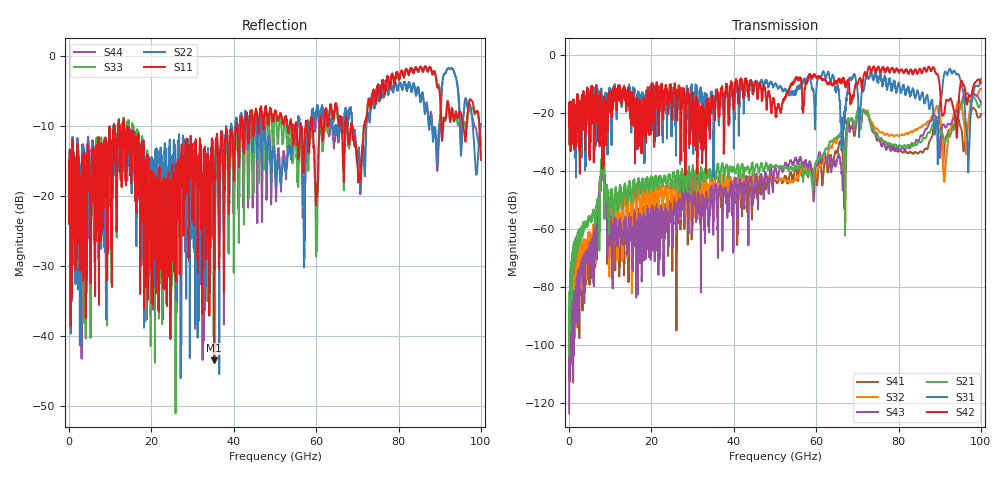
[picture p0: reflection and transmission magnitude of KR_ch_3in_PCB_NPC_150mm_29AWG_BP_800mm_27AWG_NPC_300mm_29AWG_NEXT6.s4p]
# GHz S RI R 45
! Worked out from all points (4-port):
!   4000 points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, 25 MHz to 100 GHz, reference 45 ohm
!   strongest paths, dB at 25 MHz, 25.02 GHz, 50.02 GHz, 75.03 GHz, 100 GHz:
!     S42: -21.3, -17.5, -18.0, -4.3, -9.8
!     S31: -21.3, -21.0, -10.2, -8.9, -8.4
!     S21: -103.8, -43.7, -38.2, -28.3, -17.0
!     S43: -123.6, -58.5, -39.1, -29.6, -16.4
!     S32: -108.9, -53.0, -42.7, -25.9, -11.9
!     S41: -111.4, -67.8, -43.2, -28.0, -20.5
!   lowest |S11| = -43.5 dB at 35.27 GHz (marker M1), VSWR 1.01, Z = 44.4 - j0.0041 ohm
!   |S11| at or under -10 dB: start of sweep to 10.87 GHz; 14.28 GHz to 40.62 GHz (26.34 GHz wide, 96 % of centre); 68.67 GHz to 71.56 GHz (2.899 GHz wide, 4.14 % of centre)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
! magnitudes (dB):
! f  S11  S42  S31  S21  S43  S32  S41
! 25 MHz  -16.8  -21.3  -21.3  -103.8  -123.6  -108.9  -111.4
! 8.025 GHz  -24.3  -27.6  -21.1  -40.7  -37.8  -39.3  -38.1
! 10.78 GHz  -10.7  -11.5  -11.7  -55.7  -59.8  -64.1  -59.6
! 35.27 GHz  -43.5  -17.2  -21.4  -39.5  -47.3  -41.9  -42.6
! 91.25 GHz  -8.8  -18.7  -6.0  -30.3  -24.7  -41.6  -30.1
! 96.85 GHz  -7.7  -15.2  -36.6  -15.2  -13.4  -24.4  -23.9
! 100 GHz  -14.8  -9.8  -8.4  -17.0  -16.4  -11.9  -20.5
